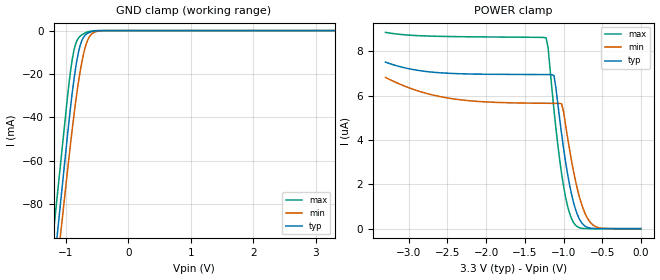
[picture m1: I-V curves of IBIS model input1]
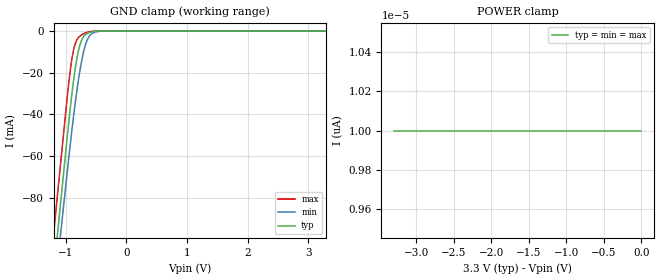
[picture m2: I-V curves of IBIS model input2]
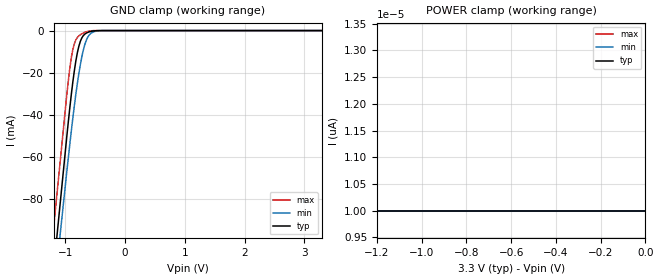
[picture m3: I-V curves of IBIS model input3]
|   Microchip Technology Inc.
|   93AA86C - 16 Kbit Microwire serial EEPROM
|   (Vcc = +1.8V to +5.5V)
|   150K Process
|   Copyright (C) 2018 Microchip Technology Inc.
[IBIS ver]   3.2
[File name]   93aa86c-i_st-3_3v.ibs
[File Rev]   1.0
[Date]   May 18, 2018
[Source]   Waveforms generated by SPICE simulation at Microchip.
   All other data taken from lab measurements at Microchip.
[Notes]   This IBIS model is for the Microchip 93AA86C device, a
   16 Kbit Microwire bus serial EEPROM manufactured on
   Microchip's 150K process, for industrial temp in a
   4.4 mm, 8-lead TSSOP package operating at 3.3V.
[Disclaimer] Unauthorized reproduction and/or distribution is
   strictly restricted. All rights reserved.
   This information is provided to you for your convenience
   and use with Microchip products only. Microchip
   disclaims all liability arising from this information
   and its use.
   THIS INFORMATION IS PROVIDED "AS IS." MICROCHIP MAKES NO
   REPRESENTATION OR WARRANTIES OF ANY KIND WHETHER EXPRESS
   OR IMPLIED, WRITTEN OR ORAL, STATUTORY OR OTHERWISE,
   RELATED TO THE INFORMATION PROVIDED TO YOU, INCLUDING
   BUT NOT LIMITED TO ITS CONDITION, QUALITY, PERFORMANCE,
   MERCHANTABILITY, NON-INFRINGEMENT, OR FITNESS FOR
   PURPOSE. MICROCHIP IS NOT LIABLE, UNDER ANY
   CIRCUMSTANCES, FOR SPECIAL, INCIDENTAL OR CONSEQUENTIAL
   DAMAGES, FOR ANY REASON WHATSOEVER.
   It is your responsibility to ensure that your
   application meets with your specifications.
|   Component 93AA86C-I/ST
[Component]   93AA86C-I/ST
[Manufacturer]   Microchip Technology Inc.
[Package]
| variable   typ   min   max
R_pkg   99.09m   85.92m   112.26m
L_pkg   2.16nH   1.55nH   2.76nH
C_pkg   0.49pF   0.43pF   0.55pF
[Pin]  signal_name   model_name
1   CS   input1
2   CLK   input2
3   DI   input3
4   DO   driver
5   VSS   GND
6   ORG   input4
7   PE   input5
8   VCC   POWER
| Models and submodels in the file (6): input1 (Input), input2 (Input), input3 (Input), driver (3-state), input4 (Input), input5 (Input)
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|   Model input1
[Model]   input1
Model_type   Input
Vinl = 0.8
Vinh = 2.0
C_comp   5.00pF   5.00pF   5.00pF
[Temperature Range]   25.00   85.00   -40.00
[Voltage Range]   3.30V   1.80V   5.50V
[Pullup Reference]   3.30V   3.30V   3.30V
[POWER Clamp Reference]   3.30V   3.30V   3.30V
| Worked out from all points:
|   GND clamp passes 1 mA (typ) near -0.64 V on its own axis
[GND_clamp]
| voltage   I(typ)   I(min)   I(max)
-3.3V     -698.8mA   -678.9mA   -676.5mA
-1.26V    -127.6mA   -139.5mA   -109.4mA
-1.175V   -103.8mA   -117.1mA   -85.74mA
-1.09V    -80mA      -94.6mA    -62.11mA
-975mV    -47.8mA    -64.19mA   -30.14mA
-900mV    -28.63mA   -45.33mA   -13.23mA
-850mV    -17.97mA   -33.8mA    -6.539mA
-800mV    -9.884mA   -23.52mA   -3.4mA
-700mV    -2.291mA   -8.439mA   -1.171mA
-600mV    -588.4uA   -1.87mA    -233.5uA
-425mV    -8.051uA   -70.28uA   -371.5nA
3.3V      10pA       10pA       10pA
[POWER_clamp]
| voltage   I(typ)   I(min)   I(max)
-3.3V     7.505uA    6.816uA    8.844uA
-2.46V    6.997uA    5.868uA    8.657uA
-1.225V   6.944uA    5.65uA     8.594uA
-1.2V     6.943uA    5.649uA    8.166uA
-1.125V   6.906uA    5.647uA    5.394uA
-1.025V   4.26uA     5.623uA    2.471uA
-950mV    2.499uA    4.142uA    1.046uA
-875mV    1.23uA     2.648uA    296.9nA
-825mV    664.2nA    1.832uA    92.72nA
-750mV    198.5nA    931.8nA    10.41nA
-625mV    11.45nA    180.5nA    10pA
0V        10pA       10pA       10pA
|   Model input2
[Model]   input2
Model_type   Input
Vinl = 0.8
Vinh = 2.0
C_comp   5.00pF   5.00pF   5.00pF
[Temperature Range]   25.00   85.00   -40.00
[Voltage Range]   3.30V   1.80V   5.50V
[Pullup Reference]   3.30V   3.30V   3.30V
[POWER Clamp Reference]   3.30V   3.30V   3.30V
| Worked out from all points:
|   GND clamp passes 1 mA (typ) near -0.64 V on its own axis
[GND_clamp]
| voltage   I(typ)   I(min)   I(max)
-3.3V     -725mA     -700mA     -708.6mA
-1.26V    -132.6mA   -144.3mA   -113.7mA
-1.175V   -107.9mA   -121.1mA   -88.95mA
-1.09V    -83.2mA    -97.98mA   -64.16mA
-975mV    -49.8mA    -66.65mA   -30.63mA
-900mV    -29.88mA   -47.23mA   -13.1mA
-850mV    -18.78mA   -35.33mA   -6.36mA
-800mV    -10.29mA   -24.69mA   -3.324mA
-700mV    -2.332mA   -8.935mA   -1.148mA
-600mV    -592.5uA   -1.955mA   -221.7uA
-425mV    -8.179uA   -72.27uA   -312.7nA
3.3V      10pA       10pA       10pA
[POWER_clamp]
| voltage   I(typ)   I(min)   I(max)
-3.3V     10pA       10pA       10pA
-3.23V    10pA       10pA       10pA
-3.16V    10pA       10pA       10pA
0V        10pA       10pA       10pA
|   Model input3
[Model]   input3
Model_type   Input
Vinl = 0.8
Vinh = 2.0
C_comp   5.00pF   5.00pF   5.00pF
[Temperature Range]   25.00   85.00   -40.00
[Voltage Range]   3.30V   1.80V   5.50V
[Pullup Reference]   3.30V   3.30V   3.30V
[POWER Clamp Reference]   3.30V   3.30V   3.30V
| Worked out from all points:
|   GND clamp passes 1 mA (typ) near -0.64 V on its own axis
[GND_clamp]
| voltage   I(typ)   I(min)   I(max)
-3.3V     -716.5mA   -689.5mA   -695.6mA
-1.26V    -131.4mA   -142.8mA   -111.4mA
-1.175V   -107mA     -120mA     -87.05mA
-1.09V    -82.64mA   -97.26mA   -62.71mA
-975mV    -49.66mA   -66.44mA   -29.77mA
-900mV    -29.95mA   -47.29mA   -12.62mA
-850mV    -18.91mA   -35.53mA   -6.134mA
-800mV    -10.43mA   -24.97mA   -3.255mA
-700mV    -2.37mA    -9.193mA   -1.131mA
-600mV    -602uA     -2.04mA    -215.6uA
-425mV    -8.622uA   -76.78uA   -289.3nA
3.3V      10pA       10pA       10pA
[POWER_clamp]
| voltage   I(typ)   I(min)   I(max)
-3.3V     10pA       1.161nA    10pA
-3.23V    10pA       10pA       10pA
-3.16V    10pA       10pA       10pA
0V        10pA       10pA       10pA
